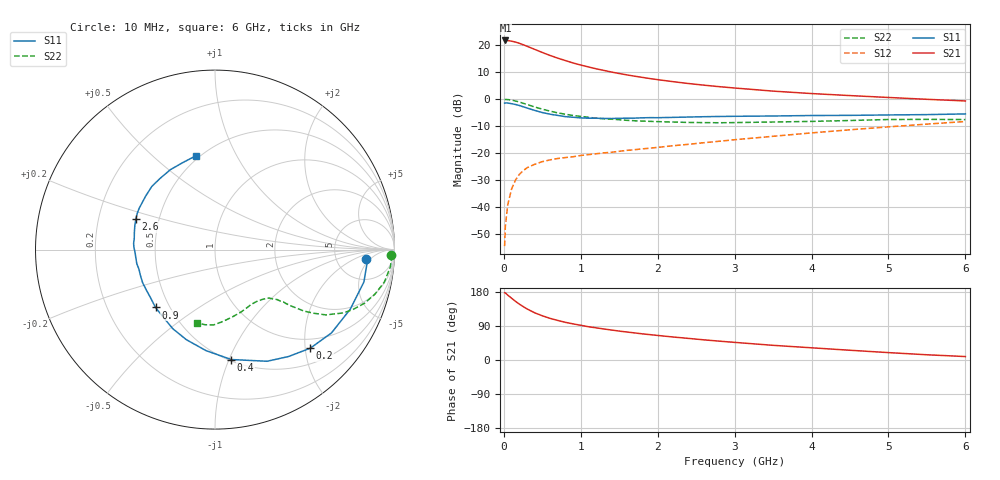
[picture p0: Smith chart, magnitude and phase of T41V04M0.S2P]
! Infineon Technologies  Discrete & RF Semiconductors
! BFR182T
! Si NPN RF Bipolar Junction Transistor in SC75
! VCE = 1 V  IC = 4 mA
! Common Emitter S-Parameters:  October  1999
# GHz  S  MA  R  50
!  f  S11  S21  S12  S22
! GHz  MAG  ANG  MAG  ANG  MAG  ANG  MAG  ANG
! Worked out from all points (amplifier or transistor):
!   36 points, 10 MHz to 6 GHz, reference 50 ohm
!   highest |S21| = 21.7 dB at 20 MHz (marker M1)
!   |S21| within 3 dB of that: start of sweep to 375.1 MHz
!   unconditionally stable (mu >= 1): 1.395 GHz to 4.409 GHz
!   at 250 MHz: K = 0.25, MSG = 23.3 dB, |S12| = -26.5 dB
!   at 1.4 GHz: K = 1.00, MAG = 14.5 dB, |S12| = -19.7 dB
!   at 6 GHz: K = 0.89, MSG = 3.8 dB, |S12| = -8.3 dB
!   S11 on the Smith chart (normalised r, x): 10 MHz: 10, -4; 200 MHz: 0.80, -2.10; 400 MHz: 0.51, -1.02; 900 MHz: 0.42, -0.34; 2.6 GHz: 0.37, +0.16; 6 GHz: 0.48, +0.70
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0.01  0.8433 -3.6  12.17 177.6  0.0019 80.6  0.9838 -1.8
0.02  0.8529 -3.4  12.2 177.0  0.0045 92.2  0.9848 -2.2
0.05  0.849 -12.3  12.14 171.3  0.011 84.5  0.9823 -5.5
0.1  0.8237 -23.7  11.82 163.2  0.0216 79.9  0.9611 -10.8
0.15  0.7979 -35.6  11.39 155.0  0.0315 71.9  0.9248 -15.6
0.2  0.7638 -46.0  10.84 147.7  0.0404 68.4  0.8854 -19.7
0.25  0.7229 -55.5  10.18 141.1  0.0472 63.5  0.84 -23.3
0.3  0.6865 -65.0  9.546 135.0  0.0536 59.7  0.7985 -26.2
0.4  0.619 -81.6  8.353 124.6  0.0622 53.9  0.7167 -30.5
0.5  0.565 -95.1  7.312 116.7  0.0697 50.7  0.6523 -32.9
0.6  0.5268 -107.6  6.439 109.9  0.0751 48.7  0.6003 -34.7
0.7  0.4997 -118.0  5.745 104.4  0.0797 47.8  0.5575 -35.7
0.8  0.4746 -127.3  5.175 99.4  0.083 46.8  0.5253 -36.6
0.9  0.4623 -135.8  4.676 95.3  0.0859 47.0  0.4981 -37.2
1.1  0.4438 -149.8  3.942 87.8  0.0941 47.5  0.4612 -38.3
1.6  0.4436 -174.4  2.811 73.8  0.1127 50.2  0.4054 -41.8
2.2  0.4596 167.7  2.106 60.7  0.1372 54.0  0.3775 -48.5
2.6  0.473 158.9  1.815 53.2  0.1562 55.8  0.3678 -54.0
3.5  0.4877 142.6  1.408 38.7  0.2054 56.9  0.3772 -67.5
4.5  0.501 127.6  1.164 25.7  0.271 54.8  0.4024 -83.5
5.5  0.5174 110.0  0.993 13.8  0.3453 50.0  0.4224 -97.7
6  0.5327 101.6  0.926 9.1  0.3855 46.6  0.4188 -104.1
